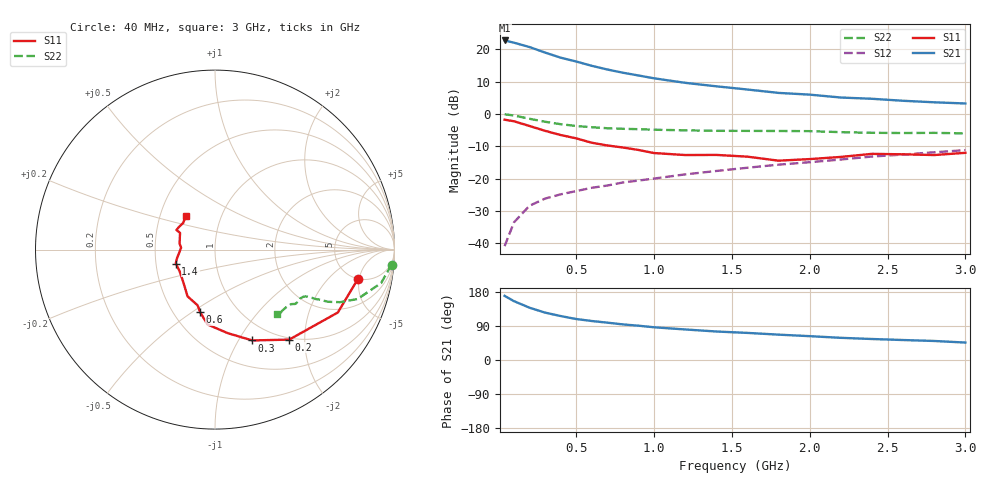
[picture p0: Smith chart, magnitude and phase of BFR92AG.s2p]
! Filename:  BFR92AG.S2P  Version:  2.0
! Philips part #: BFR92A  Date: May 1990
! Bias condition: Vce=10V, Ic=5mA
#  MHz  S  MA  R  50
! Freq  S11  S21  S12  S22  !GUM [dB]
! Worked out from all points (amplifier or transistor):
!   21 points, 40 MHz to 3 GHz, reference 50 ohm
!   highest |S21| = 22.7 dB at 40 MHz (marker M1)
!   |S21| within 3 dB of that: start of sweep to 256.1 MHz
!   unconditionally stable (mu >= 1): 1.22 GHz to 2.388 GHz; 2.44 GHz to 2.778 GHz
!   at 300 MHz: K = 0.50, MSG = 22.6 dB, |S12| = -26.2 dB
!   at 1 GHz: K = 0.97, MSG = 15.5 dB, |S12| = -20.0 dB
!   at 3 GHz: K = 0.98, MSG = 7.2 dB, |S12| = -11.2 dB
!   S11 on the Smith chart (normalised r, x): 40 MHz: 4.97, -4.80; 200 MHz: 0.97, -1.68; 300 MHz: 0.79, -1.14; 600 MHz: 0.67, -0.54; 1.4 GHz: 0.63, -0.10; 3 GHz: 0.68, +0.27
40  0.813 -11.6  13.67 169.3  0.009 82.2  0.987 -4.9
100  0.769 -27.1  12.63 155.3  0.021 74.3  0.944 -11.4
200  0.65 -50.5  10.81 138.0  0.038 68.1  0.841 -19.1
300  0.547 -67.7  8.877 125.0  0.049 63.7  0.756 -22.8
400  0.471 -81.3  7.404 116.0  0.057 62.0  0.693 -24.8
500  0.419 -95.8  6.458 108.1  0.064 61.1  0.65 -25.5
600  0.358 -103.4  5.54 102.9  0.072 62.4  0.622 -26.2
700  0.325 -107.4  4.858 98.5  0.078 64.2  0.6 -26.5
800  0.302 -120.5  4.332 93.9  0.087 64.5  0.588 -26.7
900  0.277 -126.3  3.927 90.5  0.093 65.4  0.58 -26.9
1000  0.248 -136.6  3.55 86.3  0.1 67.0  0.569 -27.3
1200  0.231 -148.8  3.023 80.6  0.116 68.8  0.557 -28.2
1400  0.232 -160.5  2.67 75.2  0.131 69.6  0.547 -29.9
1600  0.218 -166.8  2.382 71.5  0.147 71.3  0.546 -31.1
1800  0.189 176.8  2.111 66.9  0.164 72.1  0.544 -32.6
2000  0.2 170.6  1.986 62.9  0.179 72.4  0.541 -34.0
2200  0.216 154.4  1.791 58.5  0.197 72.9  0.522 -35.6
2400  0.241 153.0  1.713 55.4  0.219 72.4  0.51 -39.1
2600  0.237 147.5  1.595 52.7  0.235 72.4  0.506 -42.4
2800  0.231 139.9  1.511 50.2  0.255 72.4  0.509 -44.9
3000  0.25 130.6  1.449 46.0  0.275 71.7  0.499 -46.0
